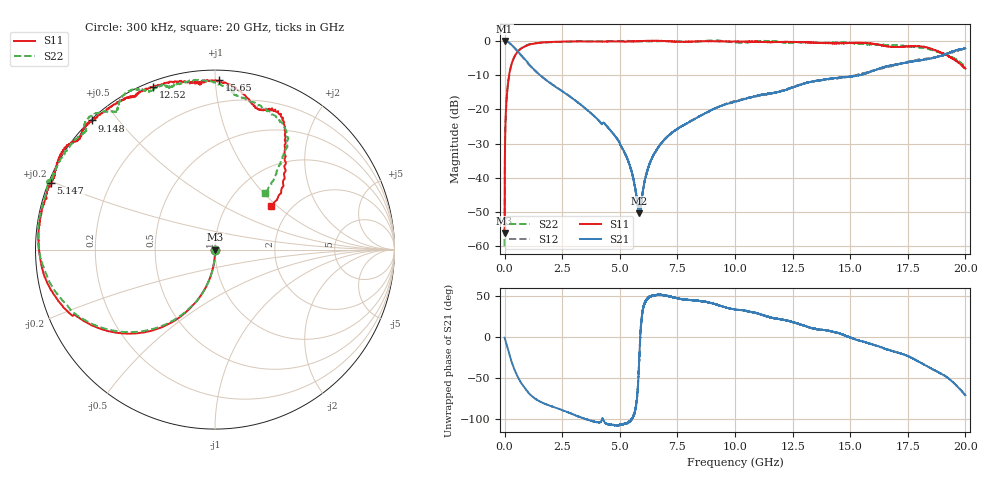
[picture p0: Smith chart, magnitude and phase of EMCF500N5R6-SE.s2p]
!EMCF500N5R6
!Johanson Technology Inc.
!www.johansontechnology.com
!Test Board Conditions:
!Substrate Type  RO4350B
!Substrate Thickness  6.6 mil
!Substrate Dk  3.66
!TL Type: GCPW
!TL Trace Width  13 mil
!TL Gap  7.5 mil
!PART MODE SINGLE ENDED (AKA BYPASS)
!DUT TOPOLOGY	SERIES-SHUNT
# MHz S  dB  R 50
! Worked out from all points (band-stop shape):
!   20001 points, 300 kHz to 20 GHz, reference 50 ohm
!   highest |S21| = 0.00 dB at 300 kHz (marker M1); lowest = -50.5 dB at 5.846 GHz (marker M2)
!   |S21| within 3 dB of the highest: start of sweep to 564.9 MHz; 19.45 GHz to end of sweep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
!   lowest |S11| = -56.2 dB at 300 kHz (marker M3), VSWR 1.00, Z = 50.2 - j0.0258 ohm
!   |S11| at or under -10 dB: start of sweep to 199.3 MHz
!   |S22| runs from -60.0 to 0.2 dB; largest |S21 - S12| = 0.027
!   S11 on the Smith chart (normalised r, x): 300 kHz: 1.00, -0.00; 5.147 GHz: 0.01, +0.19; 9.148 GHz: 0.00, +0.43; 12.52 GHz: 0.02, +0.69; 15.65 GHz: 0.06, +1.02; 20 GHz: 1.58, +0.92
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0.3  -56.19 -9.5  0.00 -0.2  0.01 -0.2  -60.03 32.4
102.298  -15.46 -100.6  -0.14 -10.4  -0.13 -10.5  -15.47 -100.6
132.298  -13.31 -103.7  -0.23 -13.5  -0.23 -13.4  -13.32 -103.6
256.296  -7.88 -116.2  -0.84 -25.6  -0.84 -25.6  -7.90 -116.7
450.293  -4.26 -131.0  -2.13 -40.7  -2.13 -40.8  -4.27 -131.9
803.288  -1.82 -149.1  -4.80 -59.1  -4.82 -59.4  -1.76 -150.7
1246.281  -0.78 -161.2  -8.13 -73.1  -8.17 -72.9  -0.69 -165.7
3334.25  -0.09 170.5  -18.75 -97.9  -18.78 -98.0  -0.05 171.0
4385.234  -0.10 162.3  -24.51 -104.9  -24.49 -104.9  -0.07 160.9
5147.223  -0.12 158.0  -31.84 -106.0  -31.90 -105.8  0.04 157.7
5497.218  -0.14 155.2  -37.87 -100.5  -37.84 -100.0  0.01 157.5
5846.212  -0.00 151.9  -50.45 -29.2  -49.89 -25.7  -0.09 157.0
6222.207  0.07 148.8  -37.35 48.2  -37.24 47.8  -0.09 155.5
6667.2  0.08 145.9  -31.15 52.1  -31.10 51.6  -0.02 151.6
9148.163  -0.04 133.7  -19.63 40.4  -19.69 40.8  0.15 133.4
10000.15  -0.14 127.0  -17.78 34.0  -17.55 34.3  -0.41 126.4
12521.11  -0.28 110.8  -13.52 18.4  -13.45 18.3  -0.40 111.5
13334.1  -0.43 100.7  -11.90 11.2  -11.84 10.8  -0.44 106.6
15650.07  -0.51 88.7  -9.48 -5.9  -9.32 -6.6  -0.90 85.7
16667.05  -1.64 75.0  -7.25 -15.3  -7.58 -15.2  -1.18 83.0
18468.02  -2.14 60.3  -5.15 -37.2  -4.99 -38.5  -2.45 57.7
20000  -8.05 38.0  -2.18 -70.5  -2.22 -69.3  -7.57 48.4
